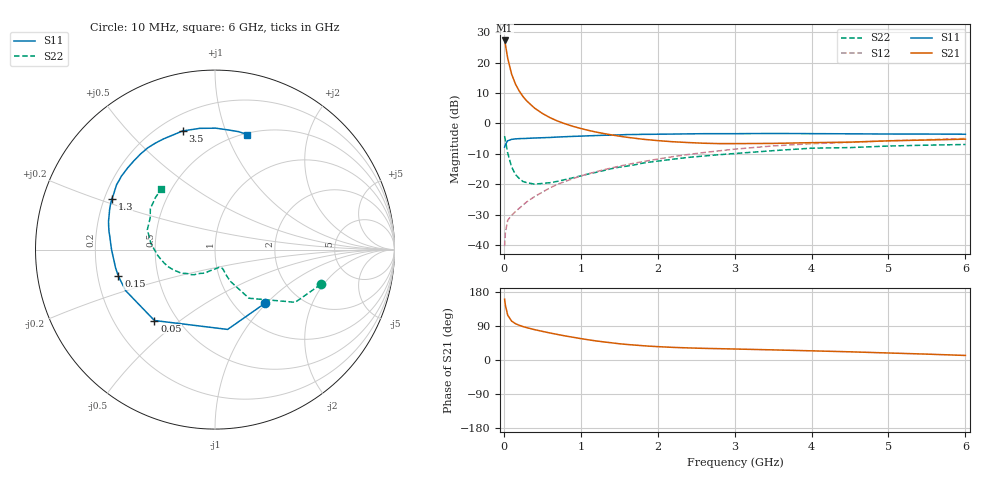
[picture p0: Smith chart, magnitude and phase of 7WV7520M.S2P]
! Infineon Technologies  Discrete & RF Semiconductors
! BFS17W
! Si NPN RF Bipolar Junction Transistor in SOT323
! VCE = 0.75 V  IC = 20 mA
! Common Emitter S-Parameters:  August  1999
# GHz  S  MA  R  50
!  f  S11  S21  S12  S22
! GHz  MAG  ANG  MAG  ANG  MAG  ANG  MAG  ANG
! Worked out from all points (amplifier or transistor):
!   36 points, 10 MHz to 6 GHz, reference 50 ohm
!   highest |S21| = 27.2 dB at 10 MHz (marker M1)
!   |S21| within 3 dB of that: start of sweep to 31.44 MHz
!   unconditionally stable (mu >= 1): start of sweep to 14.28 MHz; 39.56 MHz to end of sweep
!   at 250 MHz: K = 2.66, MAG = 10.7 dB, |S12| = -26.8 dB
!   at 1.4 GHz: K = 2.40, MAG = -1.2 dB, |S12| = -14.6 dB
!   at 6 GHz: K = 1.16, MAG = -2.6 dB, |S12| = -4.9 dB
!   S11 on the Smith chart (normalised r, x): 10 MHz: 1.37, -0.98; 50 MHz: 0.38, -0.41; 150 MHz: 0.29, -0.12; 1.3 GHz: 0.23, +0.22; 3.5 GHz: 0.29, +0.72; 6 GHz: 0.51, +1.18
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0.01  0.4088 -46.8  23.01 160.6  0.0097 70.7  0.6207 -18.2
0.02  0.4502 -81.0  19.88 144.5  0.0162 59.5  0.5347 -33.3
0.05  0.5196 -130.5  11.79 118.3  0.0258 42.7  0.3303 -55.1
0.1  0.5481 -155.4  6.523 102.9  0.031 40.6  0.1942 -64.4
0.15  0.5585 -164.6  4.46 96.0  0.0357 45.0  0.1461 -66.8
0.2  0.5635 -169.8  3.407 91.6  0.0406 49.5  0.125 -67.1
0.25  0.5659 -173.7  2.755 88.1  0.0459 52.8  0.1113 -68.8
0.3  0.5694 -176.1  2.327 85.3  0.0519 55.4  0.1067 -71.1
0.4  0.5772 179.5  1.784 80.1  0.0631 59.4  0.1011 -77.5
0.5  0.5831 176.2  1.463 75.6  0.0745 62.3  0.1038 -82.1
0.6  0.5895 173.3  1.245 71.3  0.0879 63.5  0.1067 -88.1
0.7  0.5988 170.4  1.094 67.3  0.1006 64.7  0.1125 -95.6
0.9  0.6141 165.0  0.896 60.0  0.1245 65.4  0.1288 -107.7
1.1  0.6275 159.4  0.77 53.3  0.1499 64.8  0.1485 -117.4
1.3  0.6404 153.8  0.683 47.7  0.1743 63.8  0.1692 -126.9
1.6  0.6571 146.5  0.593 41.0  0.2109 62.0  0.1996 -137.7
2.2  0.6701 132.3  0.501 33.3  0.2855 56.7  0.2595 -154.5
2.8  0.68 119.0  0.467 29.9  0.3555 49.9  0.3071 -170.1
3.5  0.6851 105.3  0.471 26.7  0.4283 41.2  0.3578 174.8
4.5  0.6765 89.6  0.494 21.6  0.4895 29.2  0.402 153.9
5.5  0.6702 78.6  0.535 15.5  0.5421 20.0  0.4406 138.8
6  0.6659 74.3  0.553 12.0  0.5669 15.4  0.4522 131.4
